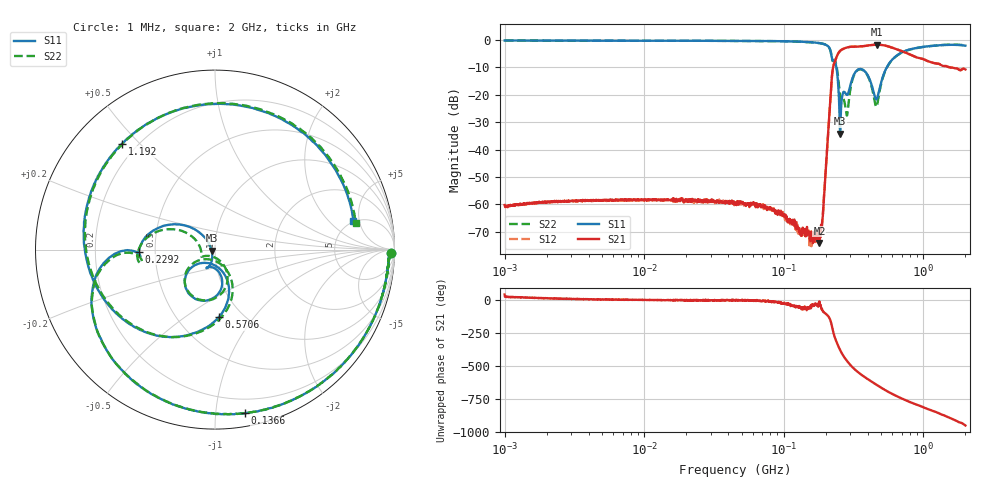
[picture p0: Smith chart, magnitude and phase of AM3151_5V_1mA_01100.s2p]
! Date/Time: Fri Jun 26 10:39:34 2020
! Network Analyzer:  Rev:
! Sweep from 1000000.0 to 2000000000.0, 1601 Points ! Power Supply: 0 V, 0 A
# HZ S DB R 50
!freq MagS11 AngS11 MagS21 AngS21 MagS12 AngS12 MagS22 AngS22
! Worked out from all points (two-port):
!   1601 points, 1 MHz to 2 GHz, reference 50 ohm
!   highest |S21| = -1.71 dB at 463 MHz (marker M1); lowest = -74.1 dB at 179.9 MHz (marker M2)
!   |S21| within 3 dB of the highest: 246.9 MHz to 753.4 MHz (506.5 MHz wide, 101 % of centre)
!   lowest |S11| = -34.2 dB at 253.3 MHz (marker M3), VSWR 1.04, Z = 48.2 - j0.644 ohm
!   |S11| at or under -10 dB: 238.1 MHz to 546.8 MHz (308.7 MHz wide, 78.6 % of centre)
!   |S22| runs from -27.6 to -0.2 dB; largest |S21 - S12| = 0.0073
!   S11 on the Smith chart (normalised r, x): 1 MHz: 53, -46; 136.6 MHz: 0.09, -1.20; 229.2 MHz: 0.40, -0.01; 570.6 MHz: 0.78, -0.69; 1.192 GHz: 0.14, +0.44; 2 GHz: 4.88, +4.10
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1000000  -0.19 -1.1  -60.25 44.9  -60.76 29.8  -0.19 -1.0
3555161  -0.25 -2.3  -58.71 10.3  -58.84 10.1  -0.24 -2.3
1.263916e7  -0.28 -7.1  -58.44 3.6  -58.57 2.7  -0.28 -7.0
4.493426e7  -0.32 -24.7  -59.30 -2.1  -59.47 1.8  -0.33 -24.6
1.365693e8  -0.65 -79.5  -68.51 -54.4  -70.23 -51.3  -0.67 -79.4
1.589914e8  -0.84 -96.1  -71.16 -30.0  -72.33 -44.7  -0.87 -96.0
1.798935e8  -1.14 -114.8  -74.13 -6.7  -72.77 -28.5  -1.13 -114.5
1.904465e8  -1.40 -126.3  -64.17 -81.6  -63.98 -78.5  -1.37 -126.1
2.1651e8  -4.11 -173.2  -19.81 -156.7  -19.82 -156.4  -4.17 -172.5
2.292112e8  -7.44 -178.4  -8.66 96.9  -8.66 96.9  -7.24 -173.0
2.532571e8  -34.21 -160.0  -3.97 -18.1  -3.98 -18.0  -20.96 166.0
2.824969e8  -20.03 -104.7  -2.77 -98.4  -2.77 -98.4  -27.57 -113.5
3.30444e8  -11.33 -92.5  -2.42 -175.2  -2.42 -175.2  -11.52 -88.0
3.958193e8  -12.57 -135.2  -2.07 123.4  -2.07 123.5  -12.75 -137.1
4.63e8  -21.59 -99.8  -1.71 76.7  -1.72 76.6  -24.26 -95.6
5.652395e8  -8.76 -84.9  -2.39 21.7  -2.40 21.7  -8.88 -81.6
5.70636e8  -8.44 -86.9  -2.46 19.3  -2.46 19.4  -8.56 -83.7
7.882285e8  -3.54 -151.1  -5.11 -50.7  -5.15 -50.6  -3.60 -151.7
9.714736e8  -2.60 169.9  -6.78 -88.1  -6.81 -87.9  -2.63 167.8
1.191643e9  -2.10 131.3  -8.45 -124.4  -8.42 -124.3  -2.09 128.4
1.547457e9  -1.77 76.3  -10.01 -174.2  -10.02 -175.0  -1.71 73.3
2e9  -2.07 11.7  -10.76 127.9  -10.93 127.1  -1.97 10.6
